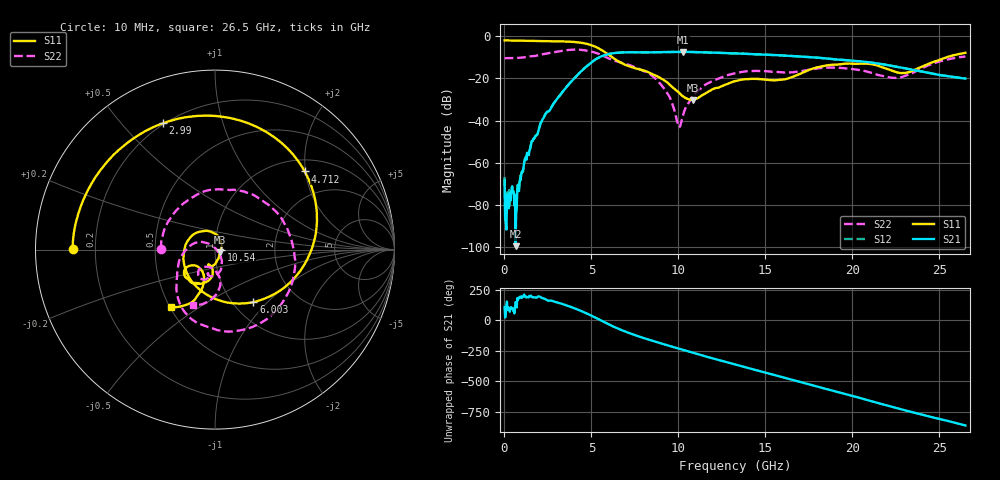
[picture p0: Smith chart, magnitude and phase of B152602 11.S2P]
!  2-Port S-parameters saved by WinCal
! VAR MeasName=S-Parameters (CALIBRATED_DATA) read from VNA (N5242A)
! VAR MeasDate=2016-1-5 16:27:00
! VAR NAME=B152602 11
! VAR FILENAME=B152602 11.S2P
! VAR DATE=2016-1-5 16:27:00
! VAR PHYS_PORTS=1,2
# Hz S DB R 50
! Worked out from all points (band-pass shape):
!   801 points, 10 MHz to 26.5 GHz, reference 50 ohm
!   highest |S21| = -7.41 dB at 10.27 GHz (marker M1); lowest = -99.5 dB at 639.1 MHz (marker M2)
!   |S21| within 3 dB of the highest: 5.356 GHz to 18.32 GHz (12.96 GHz wide, 110 % of centre)
!   lowest |S11| = -30.2 dB at 10.84 GHz (marker M3), VSWR 1.06, Z = 52.8 - j1.5 ohm
!   |S11| at or under -10 dB: 6.205 GHz to 25.42 GHz (19.21 GHz wide, 122 % of centre)
!   |S22| runs from -43.1 to -6.3 dB; largest |S21 - S12| = 0.0025
!   S11 on the Smith chart (normalised r, x): 10 MHz: 0.12, +0.00; 2.99 GHz: 0.20, +0.65; 4.712 GHz: 1.27, +1.98; 6.003 GHz: 1.23, -0.83; 10.54 GHz: 1.07, -0.01; 26.5 GHz: 0.51, -0.39
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1e7  -2.01 179.8  -68.26 108.4  -66.74 93.2  -10.47 179.5
1.755625e8  -2.02 176.3  -74.92 83.7  -72.83 85.6  -10.39 169.7
6.391375e8  -2.07 166.8  -99.48 148.5  -83.04 97.2  -10.33 142.4
1.632512e9  -2.19 146.1  -49.59 -173.3  -49.83 -173.7  -9.45 84.8
2.990125e9  -2.37 112.4  -30.15 147.9  -30.17 147.7  -7.38 8.7
4.447075e9  -3.15 55.8  -16.35 73.5  -16.35 73.5  -6.51 -71.2
4.711975e9  -3.57 41.1  -14.35 57.1  -14.36 57.1  -6.83 -84.8
5.308e9  -5.30 1.6  -10.65 15.7  -10.65 15.8  -8.02 -112.4
6.003362e9  -8.82 -53.9  -8.43 -34.4  -8.42 -34.4  -10.57 -136.5
7.129188e9  -14.16 -148.4  -7.62 -102.5  -7.61 -102.6  -13.50 -161.8
8.851038e9  -19.30 108.6  -7.56 177.0  -7.56 176.9  -21.52 149.5
9.513288e9  -23.06 70.9  -7.49 148.8  -7.49 148.8  -29.12 130.0
1.000998e10  -26.57 38.1  -7.44 127.8  -7.43 127.8  -42.72 71.5
1.027488e10  -28.51 16.8  -7.41 116.5  -7.42 116.5  -37.34 -26.2
1.053978e10  -29.73 -6.5  -7.45 105.3  -7.44 105.5  -32.08 -39.4
1.083779e10  -30.21 -27.5  -7.48 93.0  -7.49 93.1  -28.25 -46.7
1.3255e10  -21.31 -93.8  -8.15 -2.2  -8.15 -2.2  -17.52 -81.6
1.544042e10  -20.87 -111.2  -8.91 -85.6  -8.88 -85.6  -16.85 -106.1
1.769208e10  -15.43 -100.0  -10.00 -172.1  -9.97 -171.9  -15.64 -104.5
1.984439e10  -12.92 -127.6  -11.48 106.2  -11.48 105.9  -15.37 -123.4
2.209604e10  -15.80 -146.9  -13.81 17.4  -13.78 17.2  -19.49 -116.3
2.65e10  -7.86 -127.3  -20.04 -141.7  -20.02 -141.9  -9.61 -112.2
